PROGRAM MAIN

VAR CONSTANT
    cInitSource			: ST_MA_MultiArray_InitPars 
							:= ( eTypeCode := eMA_TypeCode_LREAL, nDims := 1, aDimSizes := [cBufferLength]);	
END_VAR

VAR
	(* Input *)
	nSample				: UDINT;                            
	
	(* Signal Generator *)
	fbFunctionGenerator_carrier	: FB_FunctionGenerator;			// carrier frequency generator
	fSetFrequency_carrier		: LREAL := 1000;				// Hz
	fSetAmplitude_carrier		: LREAL := 10;					// peak amplitude of carrier		
	fbFunctionGenerator_modultaor	: FB_FunctionGenerator;		// amplitude modulation part signal generator
	fSetFrequency_mod		: LREAL := 500;						// Hz
	fSetAmplitude_mod		: LREAL := 4;						// peak amplitude of amplitude modultaion
    aBuffer_carrier			: ARRAY[1..cOversamples] OF LREAL;                    
	aBuffer_modulator		: ARRAY[1..cOversamples] OF LREAL;
	
	(* Source buffers *)		
	aBuffer			    : ARRAY[1..cOversamples] OF LREAL;			
	fbSource			: FB_CMA_Source :=(	stInitPars := cInitSource, 
											nOwnID     := eID_Source, 
											aDestIDs   := [eID_PowerSpectrum, eID_PowerCepstrum],
											nResultBuffers := 5);	// Initialize source buffers
	(* Result buffers *)										
	aCepstrumResult		: ARRAY[1..cFFTResult] OF LCOMPLEX;	            // local result variable <- from sink
    fbSink_Ceps			: FB_CMA_Sink := (nOwnID := eID_Sink_Ceps);		// Initialize sink buffers
	bCalculate          : BOOL;
	aAbsCepstrumResult	: ARRAY[1..cFFTResult] OF LREAL;	
	
	aSpectrumResult		: ARRAY[1..cFFTResult] OF LREAL;	 
	fbSink_Spec         : FB_CMA_Sink := (nOwnID := eID_Sink_Spec);     
    
	(* error monitoring *)
	fbErrHist			: FB_HRErrHist;	
	
	
END_VAR


(* generate beat signal ; expected result in abs(PowerCepstrum) is peak at 2 ms = 1/500 Hz*)
ACT_SignalGenerator();


(* Call source to collect data *)
fbSource.Input1D( pDataIn 			:= ADR(aBuffer),
				  nDataInSize 		:= SIZEOF(aBuffer), 
				  eElementType 		:= eMA_TypeCode_LREAL,
				  nWorkDim 			:= 0,
				  pStartIndex		:= 0,
				  nOptionPars		:= cCMA_Option_MarkInterruption ); 
IF fbSource.bError THEN
	fbErrHist.AddError(bErr:=TRUE, hrErrCode:=fbSource.hrErrorCode, sErrSource:='MAIN.fbSource'); // error monitoring
	// ToDo: if error
END_IF


(* Push results to sink *)
fbSink_Spec.Output1D(	pDataOut 		:= ADR(aSpectrumResult), 
						nDataOutSize 	:= SIZEOF(aSpectrumResult), 
						eElementType 	:= eMA_TypeCode_LREAL, 
						nWorkDim 		:= 0,
						nElements		:= 0,
						pStartIndex 	:= 0,
						nOptionPars		:= 0,
						bNewResult		=>  );
IF fbSink_Spec.bError THEN
	fbErrHist.AddError(bErr:=TRUE, hrErrCode:=fbSink_Spec.hrErrorCode, sErrSource:='MAIN.fbSink_Spec'); // error monitoring
	// ToDo: if error
END_IF


fbSink_Ceps.Output1D(	pDataOut 		:= ADR(aCepstrumResult), 
						nDataOutSize 	:= SIZEOF(aCepstrumResult), 
						eElementType 	:= eMA_TypeCode_LCOMPLEX, 
						nWorkDim 		:= 0,
						nElements		:= 0,
						pStartIndex 	:= 0,
						nOptionPars		:= 0,
						bNewResult		=> bCalculate );
IF fbSink_Ceps.bError THEN
	fbErrHist.AddError(bErr:=TRUE, hrErrCode:=fbSink_Ceps.hrErrorCode, sErrSource:='MAIN.fbSink_Ceps'); // error monitoring
	// ToDo: if error
END_IF


IF bCalculate THEN
	// calculate squared absolute value of complex quantity
	FOR nSample := 1 TO cFFTResult DO
		// sqrt(re^2+im^2)^2
		aAbsCepstrumResult[nSample] := aCepstrumResult[nSample].re*aCepstrumResult[nSample].re + aCepstrumResult[nSample].im * aCepstrumResult[nSample].im;
	END_FOR
END_IF

ACTION ACT_SignalGenerator:
(* Input *) 

(* signal generator *)		
// generate normalised carrier signal
fbFunctionGenerator_carrier(	fFrequency 	:= fSetFrequency_carrier,
						fAmplitude 	:= 1,
						eFunction 	:= E_FunctionType.Sine,
						aSignal		:= aBuffer_carrier);
// generate normalised modulation
fbFunctionGenerator_modultaor(	fFrequency 	:= fSetFrequency_mod,
						fAmplitude 	:= 1,
						eFunction 	:= E_FunctionType.Sine,
						aSignal		:= aBuffer_modulator);
// design an amplitude modulation: A_c * sin(2*pi*f_c) * (1+A_m/A_c*sin(2*pi*fm))
FOR nSample := 1 TO cOversamples DO
	aBuffer[nSample] := fSetAmplitude_carrier*aBuffer_carrier[nSample]*(1+fSetAmplitude_mod/fSetAmplitude_carrier*aBuffer_modulator[nSample]);		
END_FOR
END_ACTION

END_PROGRAM
